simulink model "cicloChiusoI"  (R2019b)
settings: Solver=FixedStepDiscrete  StartTime=0.0  StopTime=30  FixedStep=1  RelTol=1e-3
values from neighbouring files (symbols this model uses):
  k = 0:50    [ScriptEse2.m]

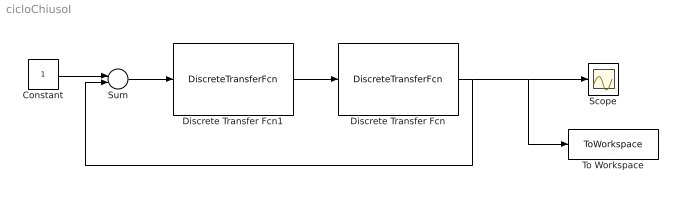
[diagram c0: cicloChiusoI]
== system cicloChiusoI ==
  Constant : Constant
  Discrete Transfer Fcn : DiscreteTransferFcn  Denominator=[1 -0.3 -0.4]
  Discrete Transfer Fcn1 : DiscreteTransferFcn  Numerator=[k 0]  Denominator=[1 -1]
  Scope : Scope
  Sum : Sum  Inputs=+-
  To Workspace : ToWorkspace  VariableName=y  SaveFormat=Timeseries  SampleTime=-1
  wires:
  Discrete Transfer Fcn/1 -> Sum/2, To Workspace/1, Scope/1
  Constant/1 -> Sum/1
  Sum/1 -> Discrete Transfer Fcn1/1
  Discrete Transfer Fcn1/1 -> Discrete Transfer Fcn/1
